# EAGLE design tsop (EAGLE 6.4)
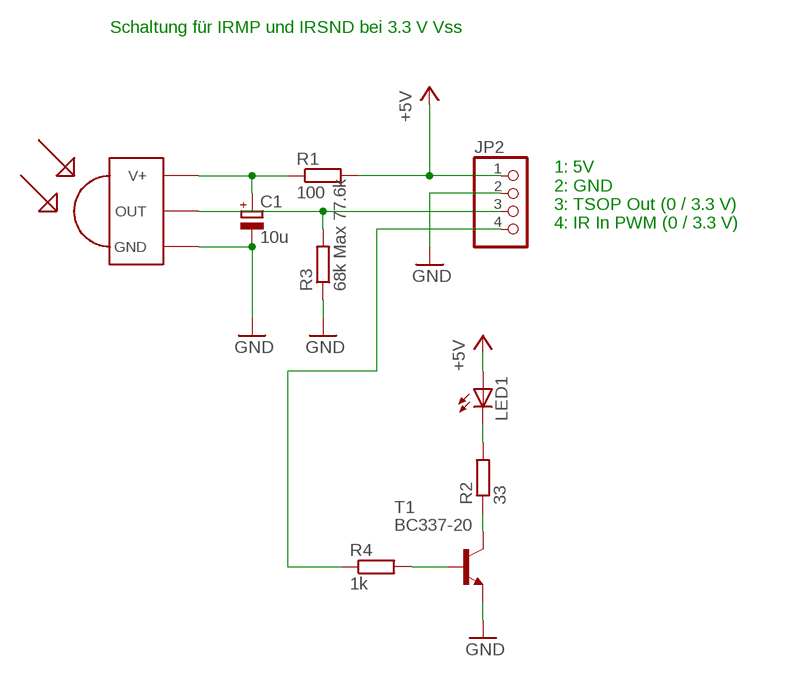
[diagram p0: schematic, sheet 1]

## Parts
C1  10u  CPOL-EUE2,5-6E  [E2,5-6E]
JP2  PINHD-1X4  [1X04]
LED1  LED5MM  [LED5MM]
R1  100  R-EU_0207/7  [0207/7]
R2  33  R-EU_0207/7  [0207/7]
R3  68k Max 77.6k  R-EU_0207/7  [0207/7]
R4  1k  R-EU_0207/10  [0207/10]
T1  BC337-20  BC337-25-NPN-TO92-CBE  [TO92-CBE]
U$1  TSOP1738  [TSOP17XX]

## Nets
+5V: JP2.1 LED1.A R1.2
GND: C1.- JP2.2 R3.1 T1.E U$1.GND
N$1: JP2.4 R4.1
N$2: C1.+ R1.1 U$1.V+
N$3: R4.2 T1.B
N$4: JP2.3 R3.2 U$1.OUT
N$5: R2.1 T1.C
N$6: LED1.K(C) R2.2

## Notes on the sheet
- Schaltung für IRMP und IRSND bei 3.3 V Vss
- 1: 5V
  2: GND
  3: TSOP Out (0 / 3.3 V)
  4: IR In PWM (0 / 3.3 V)

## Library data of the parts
C1 = rcl:CPOL-EU: POLARIZED CAPACITOR, European symbol
JP2 = pinhead:PINHD-1X4: PIN HEADER
LED1 = led:LED: LED
R1-R4 = rcl:R-EU_: RESISTOR, European symbol
T1 = transistor:*-NPN-: NPN Transistror BF959 corrected 2008.03.06
U$1 = tsop:TSOP1738: IR Receiver and Demodulator

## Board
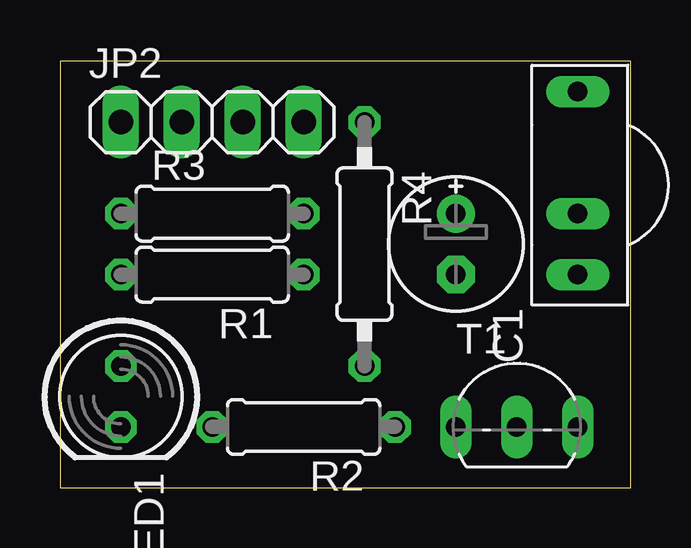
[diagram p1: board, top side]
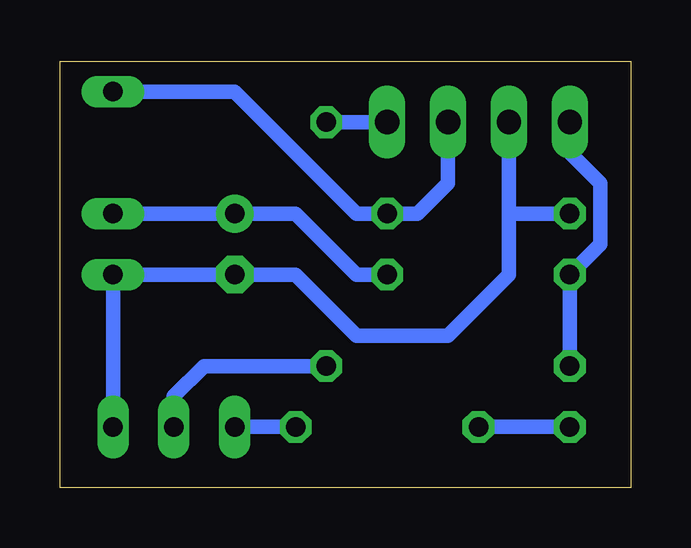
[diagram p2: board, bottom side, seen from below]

Size 23.8 x 17.77 mm. Coordinates in mm from the lower left corner, seen from the top.
Outline: 0,0 23.8,0 23.8,17.77 0,17.77 0,0
Copper layers (1*16): Top 0.035mm / dielectric 1.5mm / Bottom 0.035mm
Design rules "default": minimum track width 10mil, minimum drill 24mil, track to track 8mil, track to pad 8mil, pad to pad 8mil, via to via 8mil, smd to smd 8mil, copper to edge 40mil, drill to drill 8mil, minimum pad ring 10mil, minimum via ring 8mil, stop-mask expansion 4mil, vias tented up to drill 0mil, thermal gap 10mil

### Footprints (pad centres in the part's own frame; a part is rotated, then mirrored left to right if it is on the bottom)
E2,5-6E = drill 0.813 pad 1.575: + -1.27,0 | drill 0.813 pad 1.575 octagon: - 1.27,0
1X04 = drill 1.016 long: 1 -3.81,0; 2 -1.27,0; 3 1.27,0; 4 3.81,0
LED5MM = drill 0.813 octagon: A -1.27,0; K 1.27,0
0207/7 = drill 0.813 octagon: 1 -3.81,0; 2 3.81,0
0207/10 = drill 0.813 octagon: 1 -5.08,0; 2 5.08,0
TO92-CBE = drill 0.813 long: B 0,0; C -2.54,0; E 2.54,0
TSOP17XX = drill 0.813 long: GND -3.81,0; OUT 3.81,0; V+ -1.27,0

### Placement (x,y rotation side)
C1  16.51,10.16 270 top
JP2  6.35,15.24 0 top
LED1  2.54,3.81 270 top
R1  6.35,8.89 180 top
R2  10.16,2.54 180 top
R3  6.35,11.43 0 top
R4  12.7,10.16 270 top
T1  19.05,2.54 0 top
U$1  21.59,12.7 90 top

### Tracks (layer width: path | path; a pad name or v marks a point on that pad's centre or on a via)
+5V
  Bottom 0.61: JP2.1 2.54,13.97 1.27,12.7 1.27,10.16 R1.2 LED1.A
GND
  Bottom 0.61: T1.E U$1.GND C1.- 13.97,8.89 11.43,6.35 7.62,6.35 5.08,8.89 5.08,11.43 | 5.08,11.43 JP2.2 | R3.1 5.08,11.43
N$1
  Bottom 0.61: JP2.4 R4.1
N$2
  Bottom 0.61: U$1.V+ C1.+ 13.97,11.43 11.43,8.89 R1.1
N$3
  Bottom 0.61: T1.B 19.05,3.81 17.78,5.08 R4.2
N$4
  Bottom 0.61: JP2.3 7.62,12.7 8.89,11.43 R3.2 11.43,11.43 16.51,16.51 U$1.OUT
N$5
  Bottom 0.61: R2.1 T1.C
N$6
  Bottom 0.61: R2.2 LED1.K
